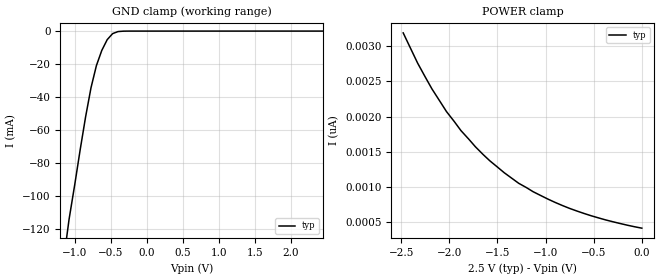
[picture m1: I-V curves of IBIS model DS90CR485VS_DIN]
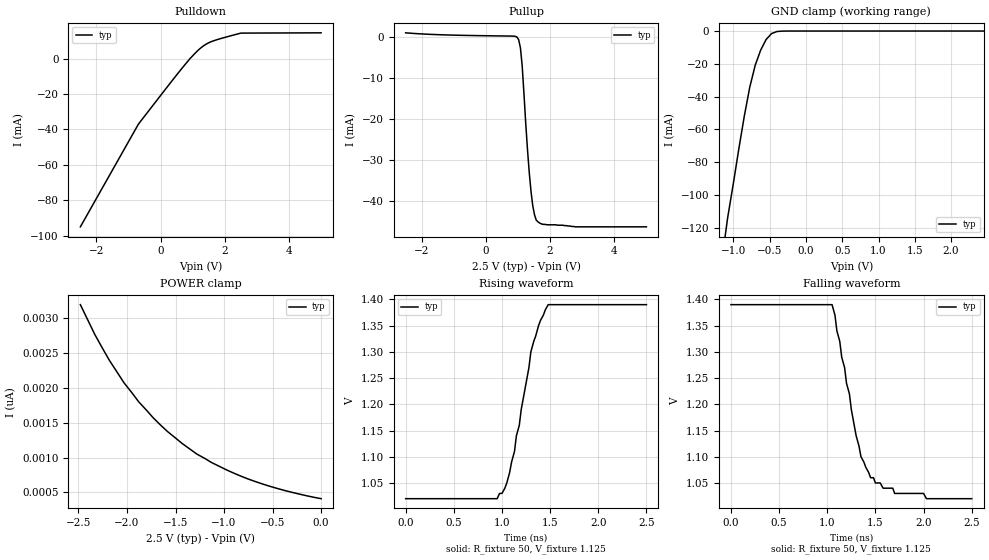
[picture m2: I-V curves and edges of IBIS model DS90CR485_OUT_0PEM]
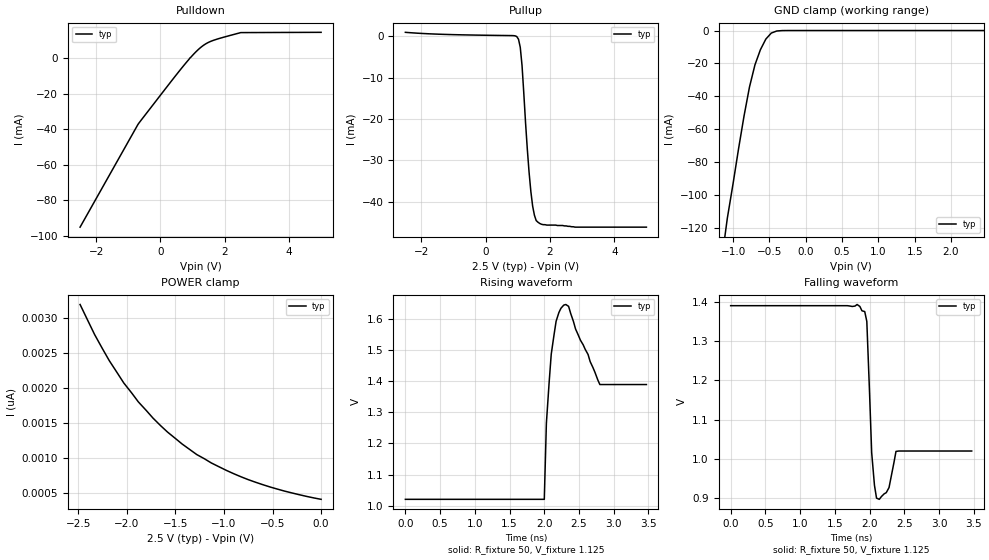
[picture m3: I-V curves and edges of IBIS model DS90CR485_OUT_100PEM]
|   National Semiconductor Corporation
|   IBIS Model of DS90CR485VS
|   133 MHz 48-Bit Channel Link Serializer
|   100-Pin TQFP Package
[IBIS Ver]   3.2
[Comment Char]   |_char
[File name]   ds90cr485vs.ibs
[File Rev]   1.0
[Date]   02/02/04
[Source]   SPICE to IBIS Translation
[Notes]
IBIS Parser Results:
Checking ds90cr485.ibs for IBIS 3.2 Compatibility...
Errors  : 0
File Passed
* Rev 1.0 Comments:
- Revision date: 02/02/04
Model Comments:
Created By: dglisic
* END Rev 1.0 Comments
[Disclaimer]
(C) Copyright National Semiconductor Corporation 2003
   All rights reserved
   National Semiconductor Corporation hereby grants
the user of this IBIS model a non-exclusive, nontransferable
license to use this IBIS model under the following terms.
Before using this IBIS model, the user should read this
license.  If the user does not accept these terms,  the
IBIS model should be returned to National within 30 days.
   The user is granted this license only to use the
IBIS model and is not granted rights to sell, load, rent,
lease or license the IBIS model in whole or in part, or in
modified form to anyone other than user. User may modify
the IBIS model to suit its specific applications but rights
to derivative works and such modifications shall belong to
National.
   This IBIS model is provided on an "AS IS" basis and
National makes absolutely no warranty with respect to the
information contained herein.NATIONAL DISCLAIMS AND CUSTOMER
WAIVES ALL WARRANTIES, EXPRESS OR IMPLIED, INCLUDING
WARRANTIES OF MERCHANTABILITY OR FITNESS FOR A PARTICULAR
PURPOSE. The entire risk as to quality and performance is
with the Customer. ACCORDINGLY, IN NO EVENT SHALL THE
COMPANY BE LIABLE FOR ANY DAMAGES, WHETHER IN CONTRACT OR
TORT,INCLUDING ANY LOST PROFITS OR OTHER INCIDENTAL,
CONSEQUENTIAL, EXEMPLARY, OR PUNITIVE DAMAGES ARISING OUT
OF THE USE OR APPLICATION OF THE IBIS model provided in
this package.Further, National reserves the right to make
changes without notice to any product herein to improve
reliability, function, or design. National does not convey
any license under patent rights or any other intellectual
property rights, including those of third parties.
   National is not obligated to provide maintenance or support
for the licensed IBIS model.
Contact National at
   ATTN:INTERFACE APPLICATIONS/IBIS MODELS
   5 Foden Road, M/S 03-03
   South Porltand, ME 04106
   (207) 541-6031
[Copyright]   (c) Copyright 2003 National Semiconductor Corp.
[Component]   DS90CR485VS
Si_location Pin
Timing_location Pin
[Manufacturer]   National Semiconductor Corp.
[Package]
|   typ   min   max
R_pkg   62.50m   58.73m   70.72m
L_pkg   2.437n   2.179n   2.917n
C_pkg   0.3272p   0.3038p   0.3789p
[Pin]   signal_name   model_name   R_pin   L_pin   C_pin
1   D7   DS90CR485VS_DIN   70.72m  2.917n   0.3789p
2   D6   DS90CR485VS_DIN   70.51m  2.771n   0.3776p
3   D5   DS90CR485VS_DIN   68.62m  2.713n   0.3658p
4   D4   DS90CR485VS_DIN   67.20m  2.650n   0.3568p
5   D3   DS90CR485VS_DIN   65.58m  2.545n   0.3467p
6   D2   DS90CR485VS_DIN   64.85m  2.496n   0.3421p
7   D1   DS90CR485VS_DIN   63.40m  2.419n   0.3328p
8   D0   DS90CR485VS_DIN   62.50m  2.437n   0.3272p
9   GND   GND   61.19m  2.376n   0.3192p
10   PLLVCC   POWER   60.16m  2.276n   0.3127p
11   GND   GND   59.45m  2.239n   0.3083p
12   PRE   DS90CR485VS_IN   58.73m  2.205n   0.3038p
13   PLLSEL   DS90CR485VS_IN   59.19m  2.179n   0.3067p
14   PLLGND   GND   58.73m  2.205n   0.3038p
15   PLLGND   GND   59.45m  2.239n   0.3083p
16   PLLVCC   POWER   60.16m  2.276n   0.3127p
17   PLLGND   GND   61.19m  2.376n   0.3192p
18   CON1   DS90CR485VS_IN   62.50m  2.437n   0.3272p
19   CON2   DS90CR485VS_IN   63.40m  2.419n   0.3328p
20   CON3   DS90CR485VS_IN   64.85m  2.496n   0.3421p
21   TSEN   NC   65.58m  2.545n   0.3467p
22   PD*   DS90CR485VS_IN   67.20m  2.650n   0.3568p
23   CON4   DS90CR485VS_IN   68.62m  2.713n   0.3658p
24   BAL   DS90CR485VS_IN   70.51m  2.771n   0.3776p
25   LVDSGND   GND   70.72m  2.917n   0.3789p
26   NC   NC   70.72m  2.917n   0.3789p
27   NC   NC   70.51m  2.771n   0.3776p
28   TxOUT7P   DS90CR485VS_OUT   68.62m  2.713n   0.3658p
29   TxOUT7M   DS90CR485VS_OUT   67.20m  2.650n   0.3568p
30   LVDSVCC   POWER   65.58m  2.545n   0.3467p
31   TxOUT6P   DS90CR485VS_OUT   64.85m  2.496n   0.3421p
32   TxOUT6M   DS90CR485VS_OUT   63.40m  2.419n   0.3328p
33   TxOUT5P   DS90CR485VS_OUT   62.50m  2.437n   0.3272p
34   TxOUT5M   DS90CR485VS_OUT   61.19m  2.376n   0.3192p
35   LVDSGND   GND   60.16m  2.276n   0.3127p
36   TxOUT4P   DS90CR485VS_OUT   59.45m  2.239n   0.3083p
37   TxOUT4M   DS90CR485VS_OUT   58.73m  2.205n   0.3038p
38   TxOUT3P   DS90CR485VS_OUT   59.19m  2.179n   0.3067p
39   TxOUT3M   DS90CR485VS_OUT   58.73m  2.205n   0.3038p
40   LVDSVCC   POWER   59.45m  2.239n   0.3083p
41   CLK1P   DS90CR485VS_OUT   60.16m  2.276n   0.3127p
42   CLK1M   DS90CR485VS_OUT   61.19m  2.376n   0.3192p
43   LVDSGND   GND   62.50m  2.437n   0.3272p
44   TxOUT2P   DS90CR485VS_OUT   63.40m  2.419n   0.3328p
45   TxOUT2M   DS90CR485VS_OUT   64.85m  2.496n   0.3421p
46   TxOUT1P   DS90CR485VS_OUT   65.58m  2.545n   0.3467p
47   TxOUT1M   DS90CR485VS_OUT   67.20m  2.650n   0.3568p
48   LVDSVCC   POWER   68.62m  2.713n   0.3658p
49   TxOUT0P   DS90CR485VS_OUT   70.51m  2.771n   0.3776p
50   TxOUT0M   DS90CR485VS_OUT   70.72m  2.917n   0.3789p
51   LVDSGND   GND   70.72m  2.917n   0.3789p
52   LVDSGND   GND   70.51m  2.771n   0.3776p
53   LVDSVCC   POWER   68.62m  2.713n   0.3658p
54   NC   NC   67.20m  2.650n   0.3568p
55   PRBS_EN   DS90CR485VS_IN   65.58m  2.545n   0.3467p
56   PAT_SEL   DS90CR485VS_IN   64.85m  2.496n   0.3421p
57   CON5   DS90CR485VS_IN   63.40m  2.419n   0.3328p
58   CON6   DS90CR485VS_IN   62.50m  2.437n   0.3272p
59   NC   NC   61.19m  2.376n   0.3192p
60   NC   NC   60.16m  2.276n   0.3127p
61   NC   NC   59.45m  2.239n   0.3083p
62   NC   NC   58.73m  2.205n   0.3038p
63   NC   NC   59.19m  2.179n   0.3067p
64   NC   NC   58.73m  2.205n   0.3038p
65   NC   NC   59.45m  2.239n   0.3083p
66   NC   NC   60.16m  2.276n   0.3127p
67   NC   NC   61.19m  2.376n   0.3192p
68   VCC   POWER   62.50m  2.437n   0.3272p
69   GND   GND   63.40m  2.419n   0.3328p
70   VCC   POWER   64.85m  2.496n   0.3421p
71   GND   GND   65.58m  2.545n   0.3467p
72   TEST1   DS90CR485VS_IN   67.20m  2.650n   0.3568p
73   TEST2   DS90CR485VS_IN   68.62m  2.713n   0.3658p
74   CON7   DS90CR485VS_IN   70.51m  2.771n   0.3776p
75   CON8   DS90CR485VS_IN   70.72m  2.917n   0.3789p
76   DS_OPT   DS90CR485VS_IN   70.72m  2.917n   0.3789p
77   GND   GND   70.51m  2.771n   0.3776p
78   NC   NC   68.62m  2.713n   0.3658p
79   VCC3   POWER   67.20m  2.650n   0.3568p
80   GND3   GND   65.58m  2.545n   0.3467p
81   D23   DS90CR485VS_DIN   64.85m  2.496n   0.3421p
82   D22   DS90CR485VS_DIN   63.40m  2.419n   0.3328p
83   D21   DS90CR485VS_DIN   62.50m  2.437n   0.3272p
84   D20   DS90CR485VS_DIN   61.19m  2.376n   0.3192p
85   D19   DS90CR485VS_DIN   60.16m  2.276n   0.3127p
86   D18   DS90CR485VS_DIN   59.45m  2.239n   0.3083p
87   CLKIN   DS90CR485VS_DIN   58.73m  2.205n   0.3038p
88   NC   NC   59.19m  2.179n   0.3067p
89   D17   DS90CR485VS_DIN   58.73m  2.205n   0.3038p
90   D16   DS90CR485VS_DIN   59.45m  2.239n   0.3083p
91   D15   DS90CR485VS_DIN   60.16m  2.276n   0.3127p
92   D14   DS90CR485VS_DIN   61.19m  2.376n   0.3192p
93   D13   DS90CR485VS_DIN   62.50m  2.437n   0.3272p
94   D12   DS90CR485VS_DIN   63.40m  2.419n   0.3328p
95   VCC   POWER   64.85m  2.496n   0.3421p
96   GND   GND   65.58m  2.545n   0.3467p
97   D11   DS90CR485VS_DIN   67.20m  2.650n   0.3568p
98   D10   DS90CR485VS_DIN   68.62m  2.713n   0.3658p
99   D9   DS90CR485VS_DIN   70.51m  2.771n   0.3776p
100   D8   DS90CR485VS_DIN   70.72m  2.917n   0.3789p
[Diff_pin]   inv_pin   vdiff   tdelay_typ   tdelay_min   tdelay_max
| The '+' pin is Diff_pin and the '-' pin is the inv_pin
28   29   NA   NA   NA   NA
31   32   NA   NA   NA   NA
33   34   NA   NA   NA   NA
36   37   NA   NA   NA   NA
38   39   NA   NA   NA   NA
41   42   NA   NA   NA   NA
44   45   NA   NA   NA   NA
46   47   NA   NA   NA   NA
49   50   NA   NA   NA   NA
[Model Selector]   DS90CR485VS_OUT
DS90CR485_OUT_100PEM   100% PEM
DS90CR485_OUT_0PEM   0% PEM
| Models and submodels in the file (4): DS90CR485VS_DIN (Input), DS90CR485VS_IN (Input), DS90CR485_OUT_0PEM (3-state), DS90CR485_OUT_100PEM (3-state)
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|   TTL DATA INPUT PINS MODEL
[Model]   DS90CR485VS_DIN
Model_type   Input
Vinh=2.0
Vinl=0.8
|   typ   min   max
C_comp   2.3pF   2.3pF   2.3pF
|   typ   min   max
[Temperature Range]   25.0   -10.0   70.0
[Voltage range]   2.5V   2.37V   2.62V
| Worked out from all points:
|   GND clamp passes 1 mA (typ) near -0.44 V on its own axis
[Power_clamp]
| Note that the [POWER_clamp] voltage table is referenced to Vcc
| and is calculated using Vtable = Vcc - Vmeasured.
|Voltage   I(typ)   I(min)   I(max)
-2.48V    3.19nA     NA         NA
-2.33V    2.76nA     NA         NA
-2.25V    2.56nA     NA         NA
-2.03V    2.07nA     NA         NA
-1.88V    1.8nA      NA         NA
-1.73V    1.57nA     NA         NA
-1.58V    1.37nA     NA         NA
-1.43V    1.2nA      NA         NA
-1.13V    930pA      NA         NA
-825mV    733pA      NA         NA
-450mV    557pA      NA         NA
0V        411pA      NA         NA
[GND_clamp]
|Voltage   I(typ)   I(min)   I(max)
-2.5V     -570mA     NA         NA
-1.15V    -137mA     NA         NA
-1.08V    -114mA     NA         NA
-850mV    -51.9mA    NA         NA
-775mV    -34.3mA    NA         NA
-700mV    -20.9mA    NA         NA
-625mV    -11.7mA    NA         NA
-550mV    -5.21mA    NA         NA
-475mV    -1.55mA    NA         NA
-400mV    -296uA     NA         NA
-325mV    -40.6uA    NA         NA
2.45V     730nA      NA         NA
|   0% Pre-emphasis LVDS OUTPUT PINS MODEL
[Model]   DS90CR485_OUT_0PEM
Model_type 3-state
Enable Active-High
Polarity Inverting
Vref=1.125
Vmeas=1.125
Rref=50   | 100 Ohms Across Outputs OUTP and OUTM
Cref=5p
C_comp   3.493pF   3.493pF   3.493pF
[Temperature Range]   25.0   -10.0   70.0
[Voltage range]   2.5V   2.37V   2.62V
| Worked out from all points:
|   slope of the pulldown table from 0 to 0.375 V, typ, clamps not added: 43 ohm
|   slope of the pullup table from 0 to 0.375 V, typ, clamps not added: 9.46 kohm
|   GND clamp passes 1 mA (typ) near -0.44 V on its own axis
|   falling waveform, R_fixture 50, V_fixture 1.125: 20-80 % time 235ps typ, NA min, NA max; typ from 1.39 V to 1.02 V
|   rising waveform, R_fixture 50, V_fixture 1.125: 20-80 % time 218ps typ, NA min, NA max; typ from 1.02 V to 1.39 V
[Pullup]
|Vtable   I(typ)   I(min)   I(max)
-2.5V     940uA      NA         NA
965mV     -75.9uA    NA         NA
1.02V     -728uA     NA         NA
1.075V    -2.69mA    NA         NA
1.13V     -7.07mA    NA         NA
1.24V     -21mA      NA         NA
1.35V     -33mA      NA         NA
1.46V     -41.1mA    NA         NA
1.57V     -44.6mA    NA         NA
1.79V     -45.6mA    NA         NA
2.78V     -46.2mA    NA         NA
5V        -46.2mA    NA         NA
[Pulldown]
|V(pulldown)   I(typ)   I(min)   I(max)
-2.5V     -95mA      NA         NA
-700mV    -37.3mA    NA         NA
719mV     -4.307mA   NA         NA
917mV     58.8uA     NA         NA
1.28V     6.397mA    NA         NA
1.61V     9.748mA    NA         NA
2.5V      14.35mA    NA         NA
5V        14.51mA    NA         NA
[GND Clamp]
-2.5V     -570mA     NA         NA
-1.15V    -137mA     NA         NA
-1.08V    -114mA     NA         NA
-850mV    -51.9mA    NA         NA
-775mV    -34.3mA    NA         NA
-700mV    -20.9mA    NA         NA
-625mV    -11.7mA    NA         NA
-550mV    -5.21mA    NA         NA
-475mV    -1.55mA    NA         NA
-400mV    -296uA     NA         NA
-325mV    -40.6uA    NA         NA
2.45V     730nA      NA         NA
[POWER Clamp]
-2.48V    3.19nA     NA         NA
-2.33V    2.76nA     NA         NA
-2.25V    2.56nA     NA         NA
-2.03V    2.07nA     NA         NA
-1.88V    1.8nA      NA         NA
-1.73V    1.57nA     NA         NA
-1.58V    1.37nA     NA         NA
-1.43V    1.2nA      NA         NA
-1.13V    930pA      NA         NA
-825mV    733pA      NA         NA
-450mV    557pA      NA         NA
0V        411pA      NA         NA
[Ramp]
dV/dt_r   210mV/.200ns   NA   NA
dV/dt_f   210mv/.250ns   NA   NA
R_load=50
[Falling Waveform]
R_fixture=50
V_fixture=1.125
| Time   V(typ)  V(min)  V(max)
0s        1.39V      NA         NA
1.05ns    1.39V      NA         NA
1.08ns    1.37V      NA         NA
1.1ns     1.34V      NA         NA
1.13ns    1.32V      NA         NA
1.3ns     1.14V      NA         NA
1.35ns    1.1V       NA         NA
1.45ns    1.06V      NA         NA
1.7ns     1.03V      NA         NA
2.5ns     1.02V      NA         NA
[Rising Waveform]
R_fixture=50
V_fixture=1.125
| Time   V(typ)  V(min)  V(max)
0s        1.02V      NA         NA
950ps     1.02V      NA         NA
1ns       1.03V      NA         NA
1.05ns    1.05V      NA         NA
1.13ns    1.11V      NA         NA
1.15ns    1.14V      NA         NA
1.3ns     1.3V       NA         NA
1.38ns    1.35V      NA         NA
1.48ns    1.39V      NA         NA
2.5ns     1.39V      NA         NA
|   100% Pre-emphasis LVDS OUTPUT PINS MODEL
[Model]   DS90CR485_OUT_100PEM
Model_type 3-state
Enable Active-High
Polarity Inverting
Vref=1.125
Vmeas=1.125
Rref=50   | 100 Ohms Across Outputs OUTP and OUTM
Cref=5p
C_comp   3.493pF   3.493pF   3.493pF
[Temperature Range]   25.0   -10.0   70.0
[Voltage range]   2.5V   2.37V   2.62V
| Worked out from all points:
|   slope of the pulldown table from 0 to 0.375 V, typ, clamps not added: 43 ohm
|   slope of the pullup table from 0 to 0.375 V, typ, clamps not added: 9.46 kohm
|   GND clamp passes 1 mA (typ) near -0.44 V on its own axis
|   falling waveform, R_fixture 50, V_fixture 1.125: 20-80 % time 47ps typ, NA min, NA max; typ from 1.39 V to 1.02 V
|   rising waveform, R_fixture 50, V_fixture 1.125: 20-80 % time 36.3ps typ, NA min, NA max; typ from 1.02 V to 1.39 V
[Pullup]
|Vtable   I(typ)   I(min)   I(max)
-2.5V     940uA      NA         NA
965mV     -75.9uA    NA         NA
1.02V     -728uA     NA         NA
1.075V    -2.69mA    NA         NA
1.13V     -7.07mA    NA         NA
1.24V     -21mA      NA         NA
1.35V     -33mA      NA         NA
1.46V     -41.1mA    NA         NA
1.57V     -44.6mA    NA         NA
1.79V     -45.6mA    NA         NA
2.78V     -46.2mA    NA         NA
5V        -46.2mA    NA         NA
[Pulldown]
|V(pulldown)   I(typ)   I(min)   I(max)
-2.5V     -95mA      NA         NA
-700mV    -37.3mA    NA         NA
719mV     -4.307mA   NA         NA
917mV     58.8uA     NA         NA
1.28V     6.397mA    NA         NA
1.61V     9.748mA    NA         NA
2.5V      14.35mA    NA         NA
5V        14.51mA    NA         NA
[GND Clamp]
-2.5V     -570mA     NA         NA
-1.15V    -137mA     NA         NA
-1.08V    -114mA     NA         NA
-850mV    -51.9mA    NA         NA
-775mV    -34.3mA    NA         NA
-700mV    -20.9mA    NA         NA
-625mV    -11.7mA    NA         NA
-550mV    -5.21mA    NA         NA
-475mV    -1.55mA    NA         NA
-400mV    -296uA     NA         NA
-325mV    -40.6uA    NA         NA
2.45V     730nA      NA         NA
[POWER Clamp]
-2.48V    3.19nA     NA         NA
-2.33V    2.76nA     NA         NA
-2.25V    2.56nA     NA         NA
-2.03V    2.07nA     NA         NA
-1.88V    1.8nA      NA         NA
-1.73V    1.57nA     NA         NA
-1.58V    1.37nA     NA         NA
-1.43V    1.2nA      NA         NA
-1.13V    930pA      NA         NA
-825mV    733pA      NA         NA
-450mV    557pA      NA         NA
0V        411pA      NA         NA
[Ramp]
dV/dt_r   210mV/.100ns   NA   NA
dV/dt_f   210mv/.1250ns   NA   NA
R_load=50
[Falling Waveform]
R_fixture=50
V_fixture=1.125
| Time   V(typ)  V(min)  V(max)
0s        1.39V      NA         NA
1.82ns    1.393V     NA         NA
1.93ns    1.375V     NA         NA
1.96ns    1.35V      NA         NA
2.03ns    1.016V     NA         NA
2.07ns    933mV      NA         NA
2.1ns     900mV      NA         NA
2.28ns    927mV      NA         NA
2.38ns    1.019V     NA         NA
3.47ns    1.02V      NA         NA
[Rising Waveform]
R_fixture=50
V_fixture=1.125
| Time   V(typ)  V(min)  V(max)
0s        1.02V      NA         NA
2ns       1.02V      NA         NA
2.03ns    1.265V     NA         NA
2.1ns     1.488V     NA         NA
2.17ns    1.594V     NA         NA
2.28ns    1.646V     NA         NA
2.35ns    1.642V     NA         NA
2.45ns    1.569V     NA         NA
2.8ns     1.39V      NA         NA
3.47ns    1.39V      NA         NA
